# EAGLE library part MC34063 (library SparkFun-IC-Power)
Jellybean switching supply controller (IC-11612, also SF)
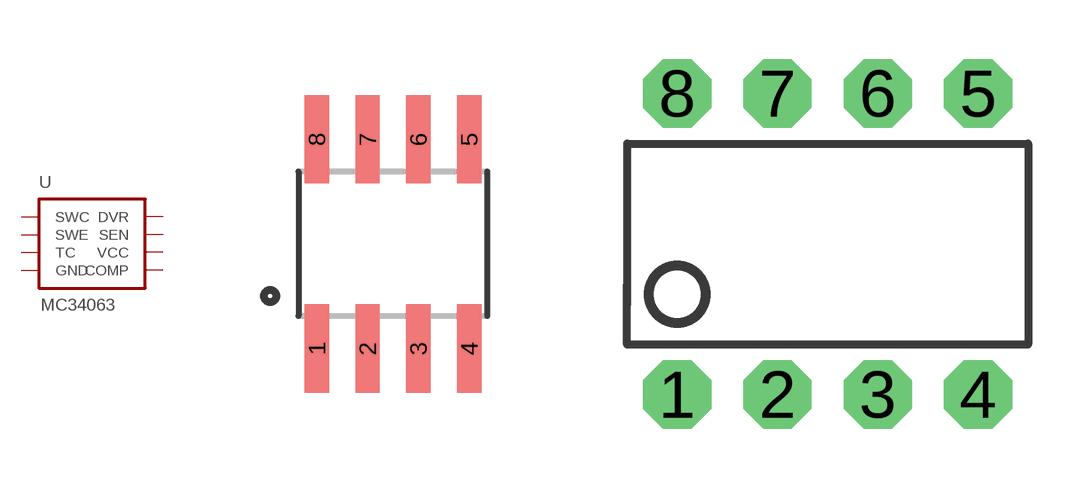
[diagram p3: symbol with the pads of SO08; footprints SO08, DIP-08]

Designator prefix U

## MC34063SMD  [SO08]
1  SWC
2  SWE
3  TC
4  GND
5  COMP
6  VCC
7  SEN
8  DVR

## MC34063DIP  [DIP-08]
Pads as for SO08

## Footprint SO08 (pad centres in mm)
Small Outline Package Fits JEDEC packages (narrow SOIC-8)
smd 0.61 x 2.21: 1 -1.905,-2.616; 2 -0.635,-2.616; 3 0.635,-2.616; 4 1.905,-2.616; 5 1.905,2.616; 6 0.635,2.616; 7 -0.635,2.616; 8 -1.905,2.616

## Footprint DIP-08 (pad centres in mm)
drill 0.813 pad 1.727 octagon: 1 -3.81,-3.81; 2 -1.27,-3.81; 3 1.27,-3.81; 4 3.81,-3.81; 5 3.81,3.81; 6 1.27,3.81; 7 -1.27,3.81; 8 -3.81,3.81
